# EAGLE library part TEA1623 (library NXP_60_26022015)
STARplug switched mode power supply controller IC The TEA1623 is a Switched Mode Power Supply (SMPS) controller IC that operates directly from rectified universal mains. It is implemented in the high voltage EZ-HV SOI process, combined with a low voltage BiCMOS process. The device includes a high voltage power switch and a circuit for start-up directly from the rectified mains voltage. A dedicated circuit for valley switching is built in, which makes a very efficient slim-line electronic power-plug concept possible. In its most basic version of application, the TEA1623 acts as a voltage source. Here, no additional secondary electronics are required. A combined voltage and current source can be realized with minimum costs for external components. Implementation of the TEA1623 renders an efficient and low cost power supply system. AAL Eindhoven MK
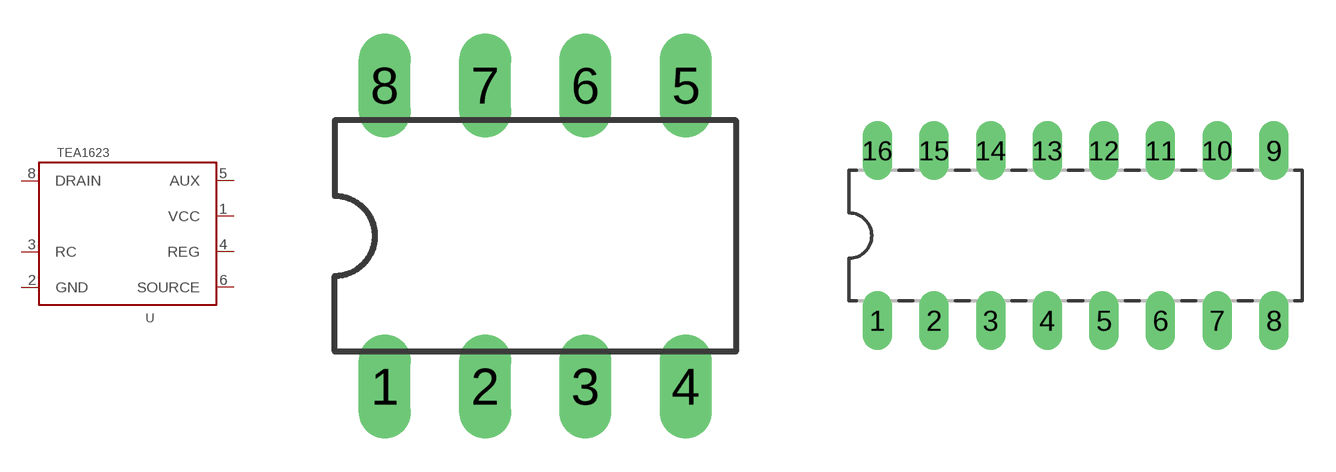
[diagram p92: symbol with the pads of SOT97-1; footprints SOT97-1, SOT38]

Designator prefix U

## TEA1623P  [SOT97-1]
1  VCC  pwr
2  GND  in
3  RC  pas
4  REG  out
5  AUX  pas
6  SOURCE  in
8  DRAIN  pas

## TEA1623PH  [SOT38]
3  VCC  pwr
4  GND  in
5  RC  pas
6  REG  out
8  GND  in
11  AUX  pas
12  SOURCE  in
14  DRAIN  pas

## Footprint SOT97-1 (pad centres in mm)
Dual In Line Package
drill 0.813 long: 1 -3.81,-3.81; 2 -1.27,-3.81; 3 1.27,-3.81; 4 3.81,-3.81; 5 3.81,3.81; 6 1.27,3.81; 7 -1.27,3.81; 8 -3.81,3.81

## Footprint SOT38 (pad centres in mm)
Dual In Line Package
drill 0.813 long: 1 -8.89,-3.81; 2 -6.35,-3.81; 3 -3.81,-3.81; 4 -1.27,-3.81; 5 1.27,-3.81; 6 3.81,-3.81; 7 6.35,-3.81; 8 8.89,-3.81; 9 8.89,3.81; 10 6.35,3.81; 11 3.81,3.81; 12 1.27,3.81; 13 -1.27,3.81; 14 -3.81,3.81; 15 -6.35,3.81; 16 -8.89,3.81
